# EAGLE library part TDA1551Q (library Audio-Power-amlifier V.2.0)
The TDA1551Q is an integrated class-B output amplifier encased in a 17-lead single-in-line plastic power package. The device contains 4 ´ 11 W single-ended (SE) or 2 ´ 22 W BTL amplifiers and is intended for use in car radio applications.
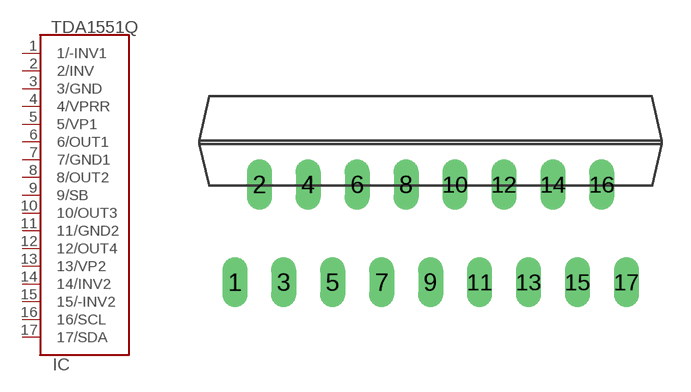
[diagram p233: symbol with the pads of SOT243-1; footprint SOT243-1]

Designator prefix IC

## TDA1551Q  [SOT243-1]
1  1/-INV1  in
2  2/INV  in
3  3/GND  pwr
4  4/VPRR  pwr
5  5/VP1  pwr
6  6/OUT1  out
7  7/GND1  pwr
8  8/OUT2  out
9  9/SB  in
10  10/OUT3  out
11  11/GND2  pwr
12  12/OUT4  out
13  13/VP2  pwr
14  14/INV2  in
15  15/-INV2  in
16  16/SCL
17  17/SDA

## Footprint SOT243-1 (pad centres in mm)
DBS17P: plastic DIL-bent-SIL power package; 17 leads (lead length 7.7 mm)
drill 0.8 long: 1 -10.16,-5.08; 2 -8.89,0; 3 -7.62,-5.08; 4 -6.35,0; 5 -5.08,-5.08; 6 -3.81,0; 7 -2.54,-5.08; 8 -1.27,0; 9 0,-5.08; 10 1.27,0; 11 2.54,-5.08; 12 3.81,0; 13 5.08,-5.08; 14 6.35,0; 15 7.62,-5.08; 16 8.89,0; 17 10.17,-5.08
